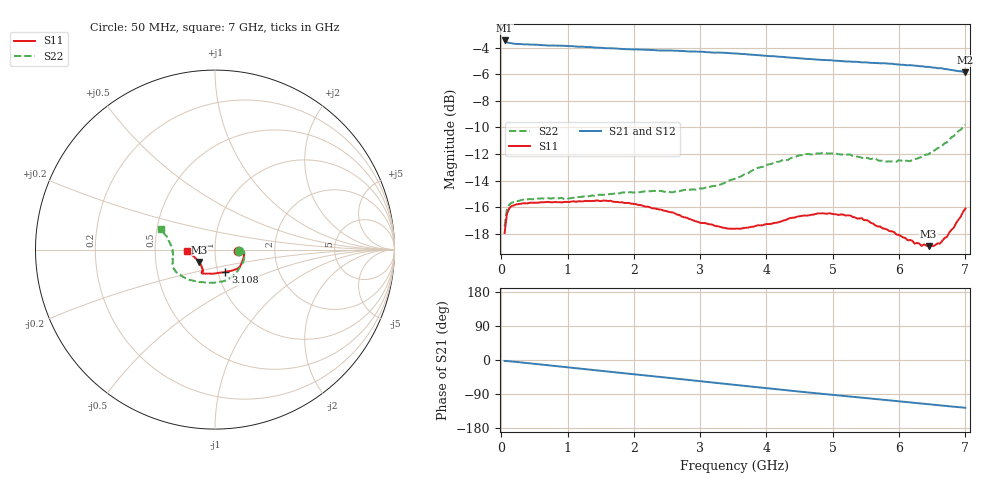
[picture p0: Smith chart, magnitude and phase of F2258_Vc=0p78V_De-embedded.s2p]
! Integrated Device Technology
! Corporate Headquarters
! 6024 Silver Creek Valley Road
! San Jose, CA 95138  USA
! Phone:  1-408-284-8200
! Toll Free:  1-800-223-1366
! Webpage:  http://www.idt.com/
! Timing and RF Division
! 515 Groton Road, Suite 102
! Westford, MA 01886-6024
! Device:  F2258
! Description: Voltage Variable RF Attenuator
! Frequency:  50.0 -  6000.00 MHz
! Package:  3x3 mm Thin QFN Plastic Package: 16 pin
! Ports:  2 RF, 2 DC
!  Pin  1  = NC
!  Pin  2  = NC
!  Pin  3  = RF2  = Port 2
!  Pin  4  = GND
!  Pin  5  = Vdd
!  Pin  6  = NC
!  Pin  7  = VCTRL
!  Pin  8  = NC
!  Pin  9  = GND
!  Pin 10  = RF1  = Port 1
!  Pin 11  = NC
!  Pin 12  = NC
!  Pin 13  = NC
!  Pin 14  = NC
!  Pin 15  = NC
!  Pin 16  = NC
! Vcntrl:  0.780 Volts
! Vdd:  +3.300 Volts
! Current:  1.130 mA
! Data:  The device was measured on a the F2258 evaluation board which has
!  individual transmission lines to the RF pins.  Data was collected
!  using a calibrated network analyzer.  The evaluation board was
!  de-embedded using a TRL calibration technique.
!  The reference plane is the edge of the package pin.
! Misc:  SN 10
!  Action Tracker AT0285
! Date Measured:  2014-12-10
! Date:  2016-01-13  MJV
! Note:
!  Integrated Device Technology supplies this data as a sample of measured
!  data at the package pin for this product.  Your particular data for this
!  product may vary.
!  Data was taken at 25 degrees C.
!  Integrated Device Technology reserves the right to change this data at anytime.
!Freq_(GHz)  S11M_(dB)  S11P_(deg)  S21M_(dB)  S21P_(deg)  S12M_(dB)  S12P_(deg)  S22M_(dB)  S22P_(deg)
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# GHz S dB R 50
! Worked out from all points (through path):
!   201 points, 50 MHz to 7 GHz, reference 50 ohm
!   highest |S21| = -3.46 dB at 50 MHz (marker M1); lowest = -5.8 dB at 7 GHz (marker M2)
!   group delay of S21, straight-line fit = 49.9 ps
!   lowest |S11| = -18.9 dB at 6.444 GHz (marker M3), VSWR 1.26, Z = 41.4 - j5.78 ohm
!   |S11| at or under -10 dB: start of sweep to end of sweep
!   |S22| runs from -17.4 to -9.8 dB; largest |S21 - S12| = 0.0032
!   S11 on the Smith chart (normalised r, x): 50 MHz: 1.29, -0.02; 3.108 GHz: 1.09, -0.28; 7 GHz: 0.73, -0.01
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0.05  -17.93 -3.1  -3.46 -2.4  -3.45 -2.4  -17.43 -3.8
0.08475  -16.50 -3.0  -3.60 -2.7  -3.59 -2.7  -16.14 -4.0
0.15425  -15.91 -4.0  -3.68 -3.8  -3.67 -3.8  -15.66 -6.4
0.606  -15.62 -14.9  -3.81 -12.2  -3.83 -12.2  -15.33 -22.3
0.9535  -15.59 -24.0  -3.87 -18.7  -3.89 -18.7  -15.41 -35.3
1.2315  -15.56 -29.3  -3.93 -23.8  -3.97 -23.8  -15.20 -44.6
1.6485  -15.51 -35.9  -4.05 -31.3  -4.07 -31.3  -15.00 -56.8
2.37825  -16.16 -46.1  -4.21 -44.4  -4.23 -44.4  -14.79 -76.7
2.58675  -16.39 -50.4  -4.22 -48.2  -4.25 -48.2  -14.87 -83.0
3.108  -17.25 -64.8  -4.35 -57.8  -4.37 -57.8  -14.47 -101.9
3.525  -17.61 -81.7  -4.44 -65.7  -4.47 -65.7  -13.85 -118.6
4.11575  -17.18 -105.2  -4.65 -76.5  -4.68 -76.5  -12.64 -139.0
4.7065  -16.55 -116.9  -4.88 -87.0  -4.89 -87.0  -12.01 -152.9
5.2625  -16.62 -120.3  -5.05 -96.5  -5.07 -96.5  -12.04 -162.1
5.43625  -16.81 -119.5  -5.11 -99.4  -5.10 -99.4  -12.27 -165.0
5.85325  -17.79 -122.6  -5.21 -106.5  -5.22 -106.5  -12.55 -173.4
6.166  -18.46 -128.8  -5.32 -111.9  -5.32 -111.9  -12.54 179.5
6.2355  -18.73 -131.9  -5.36 -113.1  -5.36 -113.1  -12.38 177.5
6.444  -18.92 -142.5  -5.45 -116.7  -5.46 -116.8  -12.03 172.3
6.61775  -18.73 -154.8  -5.54 -119.7  -5.55 -119.7  -11.48 167.5
6.722  -18.23 -161.1  -5.63 -121.6  -5.62 -121.6  -11.12 164.7
7  -16.10 -177.4  -5.85 -126.1  -5.86 -126.1  -9.79 159.1
